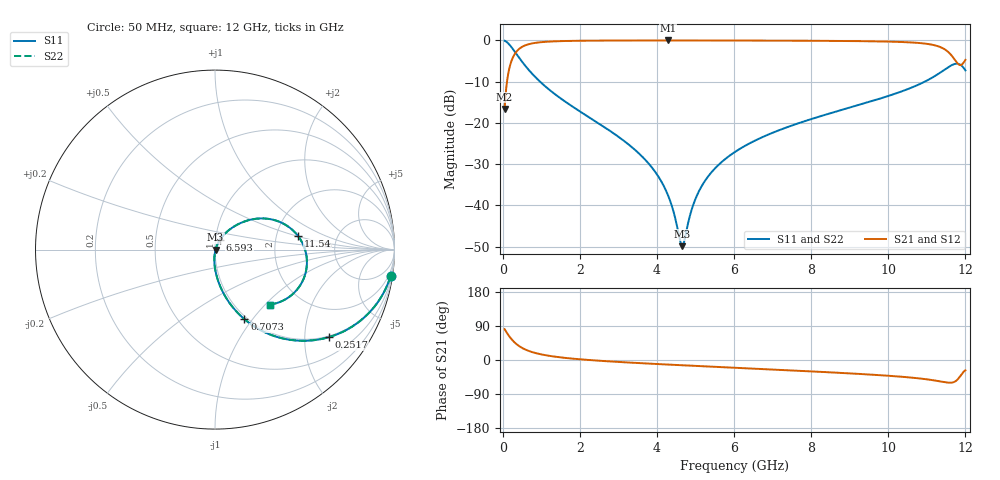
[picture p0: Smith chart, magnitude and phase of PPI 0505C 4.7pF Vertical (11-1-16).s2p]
# GHz S MA R 50
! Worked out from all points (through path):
!   1601 points, 50 MHz to 12 GHz, reference 50 ohm
!   highest |S21| = -0.03 dB at 4.285 GHz (marker M1); lowest = -16.6 dB at 50 MHz (marker M2)
!   group delay of S21, straight-line fit = 18.3 ps
!   lowest |S11| = -49.9 dB at 4.658 GHz (marker M3), VSWR 1.01, Z = 50.3 - j0.07 ohm
!   |S11| at or under -10 dB: 967 MHz to 10.95 GHz (9.982 GHz wide, 168 % of centre)
!   |S22| runs from -49.9 to -0.1 dB; largest |S21 - S12| = 0
!   S11 on the Smith chart (normalised r, x): 50 MHz: 1, -13; 251.7 MHz: 0.97, -2.62; 707.2 MHz: 0.97, -0.91; 6.593 GHz: 1.05, +0.12; 11.54 GHz: 2.65, +0.52; 12 GHz: 1.41, -1.06
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0.05  0.9891 -8.6  0.1472 81.4  0.1472 81.4  0.9891 -8.6
0.1545625  0.9082 -25.2  0.4183 64.8  0.4183 64.8  0.9082 -25.2
0.2516563  0.7993 -37.7  0.6004 52.3  0.6004 52.3  0.7993 -37.7
0.4607812  0.5853 -55.5  0.8099 34.4  0.8099 34.4  0.5853 -55.5
0.70725  0.4212 -67.1  0.9057 22.8  0.9057 22.8  0.4212 -67.1
1.177781  0.2591 -78.2  0.9642 11.5  0.9642 11.5  0.2591 -78.2
2.044156  0.1337 -87.6  0.9888 1.5  0.9888 1.5  0.1337 -87.6
3.33625  0.05141 -94.1  0.9958 -7.0  0.9958 -7.0  0.05141 -94.1
4.038312  0.02232 -93.2  0.9965 -10.8  0.9965 -10.8  0.02232 -93.2
4.284781  0.01336 -88.9  0.9966 -12.1  0.9966 -12.1  0.01336 -88.9
4.658219  0.003205 -12.5  0.9965 -13.9  0.9965 -13.9  0.003205 -12.5
4.934563  0.009922 55.2  0.9963 -15.3  0.9963 -15.3  0.009922 55.2
5.158625  0.01703 62.1  0.9961 -16.3  0.9961 -16.3  0.01703 62.1
5.524594  0.02866 64.7  0.9957 -18.1  0.9957 -18.1  0.02866 64.7
6.025  0.04446 64.6  0.9948 -20.5  0.9948 -20.5  0.04446 64.6
6.592625  0.06253 63.1  0.9935 -23.2  0.9935 -23.2  0.06253 63.1
8.019156  0.1118 57.2  0.988 -30.1  0.988 -30.1  0.1118 57.2
10.01331  0.2127 45.2  0.965 -41.6  0.965 -41.6  0.2127 45.2
10.93944  0.3146 33.5  0.9147 -50.2  0.9147 -50.2  0.3146 33.5
11.54441  0.4687 9.4  0.73 -59.6  0.73 -59.6  0.4687 9.4
11.77594  0.5211 -14.3  0.5396 -53.5  0.5396 -53.5  0.5211 -14.3
12  0.4324 -45.1  0.5788 -27.3  0.5788 -27.3  0.4324 -45.1
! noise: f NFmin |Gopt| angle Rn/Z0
0.05  0.0005235  0.9089  2.142  0.001262
1.372  0.004933  0.7285  4.777  0.00361
2.701  0.008129  0.6842  8.458  0.004965
4.031  0.01103  0.6589  12.17  0.006109
5.36  0.01388  0.6443  15.85  0.007253
6.682  0.01692  0.6392  19.45  0.008607
8.012  0.02072  0.6474  23.05  0.01072
9.341  0.02729  0.6835  26.73  0.01585
10.67  0.04966  0.7904  30.73  0.04545
12  0.2832  0.9552  34.9  1.296
